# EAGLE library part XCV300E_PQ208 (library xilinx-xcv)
xcv300e_pq208 edit this description Auto generated by make-symbol-device-package-bsdl.ulp Rev. 26 Source: xcv300e_pq208.bsd
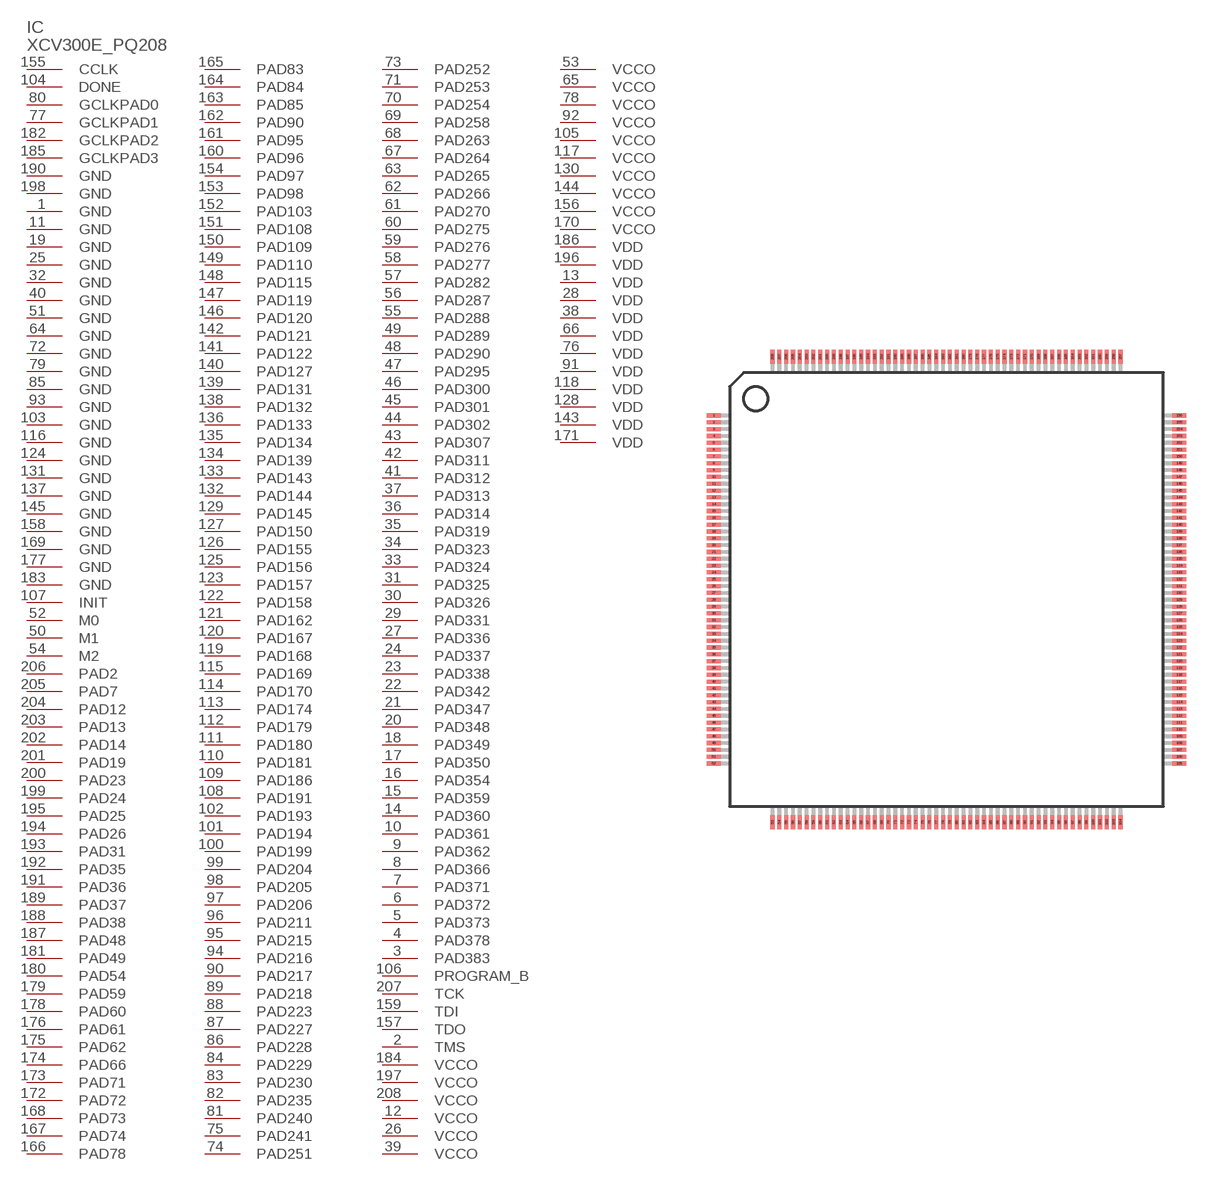
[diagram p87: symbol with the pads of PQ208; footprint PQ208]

Designator prefix IC

## XCV300E_PQ208 (OC_FARNELL: unknown; OC_NEWARK: unknown)  [PQ208]
1  GND  pwr
2  TMS  in
3  PAD383
4  PAD378
5  PAD373
6  PAD372
7  PAD371
8  PAD366
9  PAD362
10  PAD361
11  GND  pwr
12  VCCO  pwr
13  VDD  pwr
14  PAD360
15  PAD359
16  PAD354
17  PAD350
18  PAD349
19  GND  pwr
20  PAD348
21  PAD347
22  PAD342
23  PAD338
24  PAD337
25  GND  pwr
26  VCCO  pwr
27  PAD336
28  VDD  pwr
29  PAD331
30  PAD326
31  PAD325
32  GND  pwr
33  PAD324
34  PAD323
35  PAD319
36  PAD314
37  PAD313
38  VDD  pwr
39  VCCO  pwr
40  GND  pwr
41  PAD312
42  PAD311
43  PAD307
44  PAD302
45  PAD301
46  PAD300
47  PAD295
48  PAD290
49  PAD289
50  M1  in
51  GND  pwr
52  M0  in
53  VCCO  pwr
54  M2  in
55  PAD288
56  PAD287
57  PAD282
58  PAD277
59  PAD276
60  PAD275
61  PAD270
62  PAD266
63  PAD265
64  GND  pwr
65  VCCO  pwr
66  VDD  pwr
67  PAD264
68  PAD263
69  PAD258
70  PAD254
71  PAD253
72  GND  pwr
73  PAD252
74  PAD251
75  PAD241
76  VDD  pwr
77  GCLKPAD1  in
78  VCCO  pwr
79  GND  pwr
80  GCLKPAD0  in
81  PAD240
82  PAD235
83  PAD230
84  PAD229
85  GND  pwr
86  PAD228
87  PAD227
88  PAD223
89  PAD218
90  PAD217
91  VDD  pwr
92  VCCO  pwr
93  GND  pwr
94  PAD216
95  PAD215
96  PAD211
97  PAD206
98  PAD205
99  PAD204
100  PAD199
101  PAD194
102  PAD193
103  GND  pwr
104  DONE
105  VCCO  pwr
106  PROGRAM_B  in
107  INIT
108  PAD191
109  PAD186
110  PAD181
111  PAD180
112  PAD179
113  PAD174
114  PAD170
115  PAD169
116  GND  pwr
117  VCCO  pwr
118  VDD  pwr
119  PAD168
120  PAD167
121  PAD162
122  PAD158
123  PAD157
124  GND  pwr
125  PAD156
126  PAD155
127  PAD150
128  VDD  pwr
129  PAD145
130  VCCO  pwr
131  GND  pwr
132  PAD144
133  PAD143
134  PAD139
135  PAD134
136  PAD133
137  GND  pwr
138  PAD132
139  PAD131
140  PAD127
141  PAD122
142  PAD121
143  VDD  pwr
144  VCCO  pwr
145  GND  pwr
146  PAD120
147  PAD119
148  PAD115
149  PAD110
150  PAD109
151  PAD108
152  PAD103
153  PAD98
154  PAD97
155  CCLK
156  VCCO  pwr
157  TDO  out
158  GND  pwr
159  TDI  in
160  PAD96
161  PAD95
162  PAD90
163  PAD85
164  PAD84
165  PAD83
166  PAD78
167  PAD74
168  PAD73
169  GND  pwr
170  VCCO  pwr
171  VDD  pwr
172  PAD72
173  PAD71
174  PAD66
175  PAD62
176  PAD61
177  GND  pwr
178  PAD60
179  PAD59
180  PAD54
181  PAD49
182  GCLKPAD2  in
183  GND  pwr
184  VCCO  pwr
185  GCLKPAD3  in
186  VDD  pwr
187  PAD48
188  PAD38
189  PAD37
190  GND  pwr
191  PAD36
192  PAD35
193  PAD31
194  PAD26
195  PAD25
196  VDD  pwr
197  VCCO  pwr
198  GND  pwr
199  PAD24
200  PAD23
201  PAD19
202  PAD14
203  PAD13
204  PAD12
205  PAD7
206  PAD2
207  TCK  in
208  VCCO  pwr

## Footprint PQ208 (pad centres in mm)
PQ208 Auto generated by make-symbol-device-package-bsdl.ulp Rev. 26
smd 1 x 0.3: 1 -17.05,12.75; 2 -17.05,12.25; 3 -17.05,11.75; 4 -17.05,11.25; 5 -17.05,10.75; 6 -17.05,10.25; 7 -17.05,9.75; 8 -17.05,9.25; 9 -17.05,8.75; 10 -17.05,8.25; 11 -17.05,7.75; 12 -17.05,7.25; 13 -17.05,6.75; 14 -17.05,6.25; 15 -17.05,5.75; 16 -17.05,5.25; 17 -17.05,4.75; 18 -17.05,4.25; 19 -17.05,3.75; 20 -17.05,3.25; 21 -17.05,2.75; 22 -17.05,2.25; 23 -17.05,1.75; 24 -17.05,1.25; 25 -17.05,0.75; 26 -17.05,0.25; 27 -17.05,-0.25; 28 -17.05,-0.75; 29 -17.05,-1.25; 30 -17.05,-1.75; 31 -17.05,-2.25; 32 -17.05,-2.75; 33 -17.05,-3.25; 34 -17.05,-3.75; 35 -17.05,-4.25; 36 -17.05,-4.75; 37 -17.05,-5.25; 38 -17.05,-5.75; 39 -17.05,-6.25; 40 -17.05,-6.75; 41 -17.05,-7.25; 42 -17.05,-7.75; 43 -17.05,-8.25; 44 -17.05,-8.75; 45 -17.05,-9.25; 46 -17.05,-9.75; 47 -17.05,-10.25; 48 -17.05,-10.75; 49 -17.05,-11.25; 50 -17.05,-11.75; 51 -17.05,-12.25; 52 -17.05,-12.75; 105 17.05,-12.75; 106 17.05,-12.25; 107 17.05,-11.75; 108 17.05,-11.25; 109 17.05,-10.75; 110 17.05,-10.25; 111 17.05,-9.75; 112 17.05,-9.25; 113 17.05,-8.75; 114 17.05,-8.25; 115 17.05,-7.75; 116 17.05,-7.25; 117 17.05,-6.75; 118 17.05,-6.25; 119 17.05,-5.75; 120 17.05,-5.25; 121 17.05,-4.75; 122 17.05,-4.25; 123 17.05,-3.75; 124 17.05,-3.25; 125 17.05,-2.75; 126 17.05,-2.25; 127 17.05,-1.75; 128 17.05,-1.25; 129 17.05,-0.75; 130 17.05,-0.25; 131 17.05,0.25; 132 17.05,0.75; 133 17.05,1.25; 134 17.05,1.75; 135 17.05,2.25; 136 17.05,2.75; 137 17.05,3.25; 138 17.05,3.75; 139 17.05,4.25; 140 17.05,4.75; 141 17.05,5.25; 142 17.05,5.75; 143 17.05,6.25; 144 17.05,6.75; 145 17.05,7.25; 146 17.05,7.75; 147 17.05,8.25; 148 17.05,8.75; 149 17.05,9.25; 150 17.05,9.75; 151 17.05,10.25; 152 17.05,10.75; 153 17.05,11.25; 154 17.05,11.75; 155 17.05,12.25; 156 17.05,12.75
smd 0.3 x 1: 53 -12.75,-17.05; 54 -12.25,-17.05; 55 -11.75,-17.05; 56 -11.25,-17.05; 57 -10.75,-17.05; 58 -10.25,-17.05; 59 -9.75,-17.05; 60 -9.25,-17.05; 61 -8.75,-17.05; 62 -8.25,-17.05; 63 -7.75,-17.05; 64 -7.25,-17.05; 65 -6.75,-17.05; 66 -6.25,-17.05; 67 -5.75,-17.05; 68 -5.25,-17.05; 69 -4.75,-17.05; 70 -4.25,-17.05; 71 -3.75,-17.05; 72 -3.25,-17.05; 73 -2.75,-17.05; 74 -2.25,-17.05; 75 -1.75,-17.05; 76 -1.25,-17.05; 77 -0.75,-17.05; 78 -0.25,-17.05; 79 0.25,-17.05; 80 0.75,-17.05; 81 1.25,-17.05; 82 1.75,-17.05; 83 2.25,-17.05; 84 2.75,-17.05; 85 3.25,-17.05; 86 3.75,-17.05; 87 4.25,-17.05; 88 4.75,-17.05; 89 5.25,-17.05; 90 5.75,-17.05; 91 6.25,-17.05; 92 6.75,-17.05; 93 7.25,-17.05; 94 7.75,-17.05; 95 8.25,-17.05; 96 8.75,-17.05; 97 9.25,-17.05; 98 9.75,-17.05; 99 10.25,-17.05; 100 10.75,-17.05; 101 11.25,-17.05; 102 11.75,-17.05; 103 12.25,-17.05; 104 12.75,-17.05; 157 12.75,17.05; 158 12.25,17.05; 159 11.75,17.05; 160 11.25,17.05; 161 10.75,17.05; 162 10.25,17.05; 163 9.75,17.05; 164 9.25,17.05; 165 8.75,17.05; 166 8.25,17.05; 167 7.75,17.05; 168 7.25,17.05; 169 6.75,17.05; 170 6.25,17.05; 171 5.75,17.05; 172 5.25,17.05; 173 4.75,17.05; 174 4.25,17.05; 175 3.75,17.05; 176 3.25,17.05; 177 2.75,17.05; 178 2.25,17.05; 179 1.75,17.05; 180 1.25,17.05; 181 0.75,17.05; 182 0.25,17.05; 183 -0.25,17.05; 184 -0.75,17.05; 185 -1.25,17.05; 186 -1.75,17.05; 187 -2.25,17.05; 188 -2.75,17.05; 189 -3.25,17.05; 190 -3.75,17.05; 191 -4.25,17.05; 192 -4.75,17.05; 193 -5.25,17.05; 194 -5.75,17.05; 195 -6.25,17.05; 196 -6.75,17.05; 197 -7.25,17.05; 198 -7.75,17.05; 199 -8.25,17.05; 200 -8.75,17.05; 201 -9.25,17.05; 202 -9.75,17.05; 203 -10.25,17.05; 204 -10.75,17.05; 205 -11.25,17.05; 206 -11.75,17.05; 207 -12.25,17.05; 208 -12.75,17.05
